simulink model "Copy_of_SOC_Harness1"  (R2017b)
settings: Solver=FixedStepDiscrete  StartTime=0.0  StopTime=2  FixedStep=0.01  RelTol=1e-3  EnableMultiTasking=on
undefined symbols (not defined in the file): sigbuilder_block

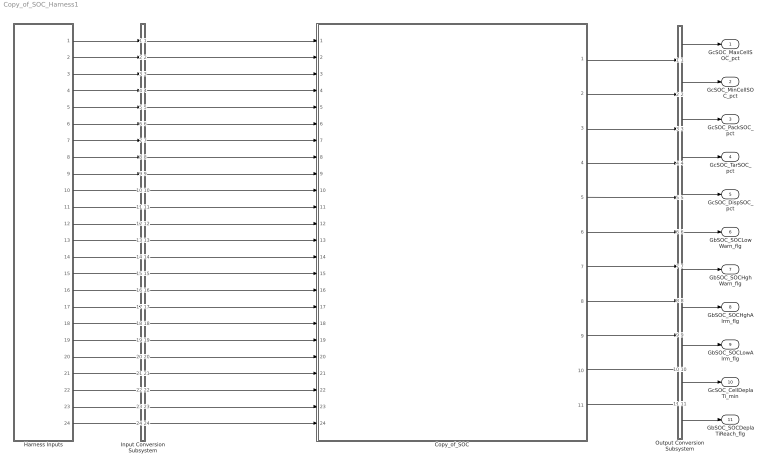
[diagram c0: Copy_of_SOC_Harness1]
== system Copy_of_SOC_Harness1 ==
  Copy_of_SOC : ModelReference  ModelNameDialog=Copy_of_SOC  SimulationMode=Normal  ModelReferenceVersion='M110C113'
  Harness Inputs : Subsystem  Tag=STV Subsys  LoadFcn=sigbuilder_block('load');  StartFcn=sigbuilder_block('start');  StopFcn=sigbuilder_block('stop');  ClipboardFcn=sigbuilder_block('clipboard');  mask(Sigbuilder block){tuvar=[0:10]}
      mask init:
      | if ~strcmp(get_param(bdroot(gcb),'SimulationStatus'),'stopped'),tuvar = sigbuilder_block('maskInit'); end
  Input Conversion Subsystem : Subsystem  Tag=__SLT_ICS__  Description=Signal spec. and routing
  Output Conversion Subsystem : Subsystem  Tag=__SLT_OCS__  Description=Signal spec. and routing
  GcSOC_MaxCellSOC_pct : Outport  OutDataTypeStr=single  PortDimensions=[1]
  GcSOC_MinCellSOC_pct : Outport  Port=2  OutDataTypeStr=single  PortDimensions=[1]
  GcSOC_PackSOC_pct : Outport  Port=3  OutDataTypeStr=single  PortDimensions=[1]
  GcSOC_TarSOC_pct : Outport  Port=4  OutDataTypeStr=single  PortDimensions=[1]
  GcSOC_DispSOC_pct : Outport  Port=5  OutDataTypeStr=single  PortDimensions=[1]
  GbSOC_SOCLowWarn_flg : Outport  Port=6  OutDataTypeStr=boolean  PortDimensions=[1]
  GbSOC_SOCHghWarn_flg : Outport  Port=7  OutDataTypeStr=boolean  PortDimensions=[1]
  GbSOC_SOCHghAlrm_flg : Outport  Port=8  OutDataTypeStr=boolean  PortDimensions=[1]
  GbSOC_SOCLowAlrm_flg : Outport  Port=9  OutDataTypeStr=boolean  PortDimensions=[1]
  GcSOC_CellDeplaTi_min : Outport  Port=10  OutDataTypeStr=uint32  PortDimensions=[1]
  GbSOC_SOCDeplaTiReach_flg : Outport  Port=11  OutDataTypeStr=boolean  PortDimensions=[1]
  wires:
  Harness Inputs/1(GcHDP_PackCrnt_A) -> Input Conversion Subsystem/1(Inport_1)
  Harness Inputs/2(GcHDP_PackVolt_V) -> Input Conversion Subsystem/2(Inport_2)
  Harness Inputs/3(GbACC_ACChrgFinish_flg) -> Input Conversion Subsystem/3(Inport_3)
  Harness Inputs/4(GbDCC_DCChrgFinish_flg) -> Input Conversion Subsystem/4(Inport_4)
  Harness Inputs/5(GcRTC_SleepTime_min) -> Input Conversion Subsystem/5(Inport_5)
  Harness Inputs/6(GcCDP_MaxCellVolt_mV) -> Input Conversion Subsystem/6(Inport_6)
  Harness Inputs/7(GcCDP_MinCellVolt_mV) -> Input Conversion Subsystem/7(Inport_7)
  Harness Inputs/8(GcCDP_MinCellTemp_C) -> Input Conversion Subsystem/8(Inport_8)
  Harness Inputs/9(GbCDP_SumCellVoltVld_flg) -> Input Conversion Subsystem/9(Inport_9)
  Harness Inputs/10(GeMSM_BMUState_enum) -> Input Conversion Subsystem/10(Inport_10)
  Harness Inputs/11(GbNDP_ReadMaxCellSOCVld_flg) -> Input Conversion Subsystem/11(Inport_11)
  Harness Inputs/12(GbNDP_ReadMinCellSOCVld_flg) -> Input Conversion Subsystem/12(Inport_12)
  Harness Inputs/13(GbNDP_ReadMaxCellVoltVld_flg) -> Input Conversion Subsystem/13(Inport_13)
  Harness Inputs/14(GbNDP_ReadMinCellVoltVld_flg) -> Input Conversion Subsystem/14(Inport_14)
  Harness Inputs/15(GcSOH_CurrBatCap_Ah) -> Input Conversion Subsystem/15(Inport_15)
  Harness Inputs/16(GbUDS_MnlSOCCorrd_flg) -> Input Conversion Subsystem/16(Inport_16)
  Harness Inputs/17(GeCTC_CtrCtlConnMode_enum) -> Input Conversion Subsystem/17(Inport_17)
  Harness Inputs/18(GbNDP_ReadDispSOCVld_flg) -> Input Conversion Subsystem/18(Inport_18)
  Harness Inputs/19(GbHDP_PackCrntVld_flg) -> Input Conversion Subsystem/19(Inport_19)
  Harness Inputs/20(GbDCC_ChrgSt2StepChrg_flg) -> Input Conversion Subsystem/20(Inport_20)
  Harness Inputs/21(GbACC_ChrgSt2StepChrg_flg) -> Input Conversion Subsystem/21(Inport_21)
  Harness Inputs/22(GcADP_YearSet_Yr) -> Input Conversion Subsystem/22(Inport_22)
  Harness Inputs/23(GbISP_TF37FTiout_flg) -> Input Conversion Subsystem/23(Inport_23)
  Harness Inputs/24(GeUDS_CapSel_enum) -> Input Conversion Subsystem/24(Inport_24)
  Output Conversion Subsystem/1(Outport_1) -> GcSOC_MaxCellSOC_pct/1
  Output Conversion Subsystem/2(Outport_2) -> GcSOC_MinCellSOC_pct/1
  Output Conversion Subsystem/3(Outport_3) -> GcSOC_PackSOC_pct/1
  Output Conversion Subsystem/4(Outport_4) -> GcSOC_TarSOC_pct/1
  Output Conversion Subsystem/5(Outport_5) -> GcSOC_DispSOC_pct/1
  Output Conversion Subsystem/6(Outport_6) -> GbSOC_SOCLowWarn_flg/1
  Output Conversion Subsystem/7(Outport_7) -> GbSOC_SOCHghWarn_flg/1
  Output Conversion Subsystem/8(Outport_8) -> GbSOC_SOCHghAlrm_flg/1
  Output Conversion Subsystem/9(Outport_9) -> GbSOC_SOCLowAlrm_flg/1
  Output Conversion Subsystem/10(Outport_10) -> GcSOC_CellDeplaTi_min/1
  Output Conversion Subsystem/11(Outport_11) -> GbSOC_SOCDeplaTiReach_flg/1
  Input Conversion Subsystem/1(Outport_1) -> Copy_of_SOC/1
  Input Conversion Subsystem/2(Outport_2) -> Copy_of_SOC/2
  Input Conversion Subsystem/3(Outport_3) -> Copy_of_SOC/3
  Input Conversion Subsystem/4(Outport_4) -> Copy_of_SOC/4
  Input Conversion Subsystem/5(Outport_5) -> Copy_of_SOC/5
  Input Conversion Subsystem/6(Outport_6) -> Copy_of_SOC/6
  Input Conversion Subsystem/7(Outport_7) -> Copy_of_SOC/7
  Input Conversion Subsystem/8(Outport_8) -> Copy_of_SOC/8
  Input Conversion Subsystem/9(Outport_9) -> Copy_of_SOC/9
  Input Conversion Subsystem/10(Outport_10) -> Copy_of_SOC/10
  Input Conversion Subsystem/11(Outport_11) -> Copy_of_SOC/11
  Input Conversion Subsystem/12(Outport_12) -> Copy_of_SOC/12
  Input Conversion Subsystem/13(Outport_13) -> Copy_of_SOC/13
  Input Conversion Subsystem/14(Outport_14) -> Copy_of_SOC/14
  Input Conversion Subsystem/15(Outport_15) -> Copy_of_SOC/15
  Input Conversion Subsystem/16(Outport_16) -> Copy_of_SOC/16
  Input Conversion Subsystem/17(Outport_17) -> Copy_of_SOC/17
  Input Conversion Subsystem/18(Outport_18) -> Copy_of_SOC/18
  Input Conversion Subsystem/19(Outport_19) -> Copy_of_SOC/19
  Input Conversion Subsystem/20(Outport_20) -> Copy_of_SOC/20
  Input Conversion Subsystem/21(Outport_21) -> Copy_of_SOC/21
  Input Conversion Subsystem/22(Outport_22) -> Copy_of_SOC/22
  Input Conversion Subsystem/23(Outport_23) -> Copy_of_SOC/23
  Input Conversion Subsystem/24(Outport_24) -> Copy_of_SOC/24
  Copy_of_SOC/1 -> Output Conversion Subsystem/1(Inport_1)
  Copy_of_SOC/2 -> Output Conversion Subsystem/2(Inport_2)
  Copy_of_SOC/3 -> Output Conversion Subsystem/3(Inport_3)
  Copy_of_SOC/4 -> Output Conversion Subsystem/4(Inport_4)
  Copy_of_SOC/5 -> Output Conversion Subsystem/5(Inport_5)
  Copy_of_SOC/6 -> Output Conversion Subsystem/6(Inport_6)
  Copy_of_SOC/7 -> Output Conversion Subsystem/7(Inport_7)
  Copy_of_SOC/8 -> Output Conversion Subsystem/8(Inport_8)
  Copy_of_SOC/9 -> Output Conversion Subsystem/9(Inport_9)
  Copy_of_SOC/10 -> Output Conversion Subsystem/10(Inport_10)
  Copy_of_SOC/11 -> Output Conversion Subsystem/11(Inport_11)

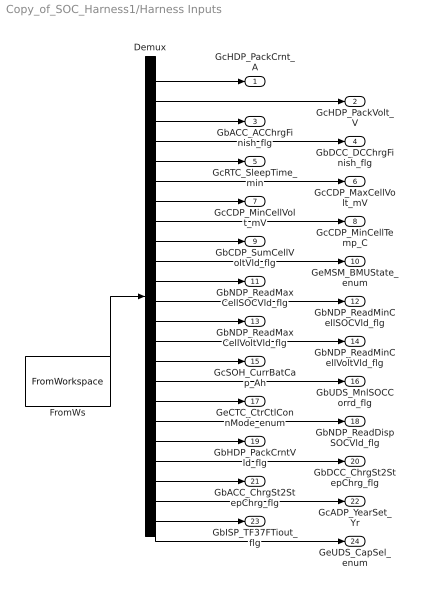
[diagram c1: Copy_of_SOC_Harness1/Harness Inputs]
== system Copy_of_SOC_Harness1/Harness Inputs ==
  Demux : Demux  Tag=STV Demux  Outputs=24
  FromWs : FromWorkspace  Tag=STV FromWs  VariableName=tuvar  SampleTime=0
  GcHDP_PackCrnt_A : Outport  Tag=STV Outport
  GcHDP_PackVolt_V : Outport  Tag=STV Outport  Port=2
  GbACC_ACChrgFinish_flg : Outport  Tag=STV Outport  Port=3
  GbDCC_DCChrgFinish_flg : Outport  Tag=STV Outport  Port=4
  GcRTC_SleepTime_min : Outport  Tag=STV Outport  Port=5
  GcCDP_MaxCellVolt_mV : Outport  Tag=STV Outport  Port=6
  GcCDP_MinCellVolt_mV : Outport  Tag=STV Outport  Port=7
  GcCDP_MinCellTemp_C : Outport  Tag=STV Outport  Port=8
  GbCDP_SumCellVoltVld_flg : Outport  Tag=STV Outport  Port=9
  GeMSM_BMUState_enum : Outport  Tag=STV Outport  Port=10
  GbNDP_ReadMaxCellSOCVld_flg : Outport  Tag=STV Outport  Port=11
  GbNDP_ReadMinCellSOCVld_flg : Outport  Tag=STV Outport  Port=12
  GbNDP_ReadMaxCellVoltVld_flg : Outport  Tag=STV Outport  Port=13
  GbNDP_ReadMinCellVoltVld_flg : Outport  Tag=STV Outport  Port=14
  GcSOH_CurrBatCap_Ah : Outport  Tag=STV Outport  Port=15
  GbUDS_MnlSOCCorrd_flg : Outport  Tag=STV Outport  Port=16
  GeCTC_CtrCtlConnMode_enum : Outport  Tag=STV Outport  Port=17
  GbNDP_ReadDispSOCVld_flg : Outport  Tag=STV Outport  Port=18
  GbHDP_PackCrntVld_flg : Outport  Tag=STV Outport  Port=19
  GbDCC_ChrgSt2StepChrg_flg : Outport  Tag=STV Outport  Port=20
  GbACC_ChrgSt2StepChrg_flg : Outport  Tag=STV Outport  Port=21
  GcADP_YearSet_Yr : Outport  Tag=STV Outport  Port=22
  GbISP_TF37FTiout_flg : Outport  Tag=STV Outport  Port=23
  GeUDS_CapSel_enum : Outport  Tag=STV Outport  Port=24
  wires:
  FromWs/1 -> Demux/1
  Demux/1 -> GcHDP_PackCrnt_A/1
  Demux/2 -> GcHDP_PackVolt_V/1
  Demux/3 -> GbACC_ACChrgFinish_flg/1
  Demux/4 -> GbDCC_DCChrgFinish_flg/1
  Demux/5 -> GcRTC_SleepTime_min/1
  Demux/6 -> GcCDP_MaxCellVolt_mV/1
  Demux/7 -> GcCDP_MinCellVolt_mV/1
  Demux/8 -> GcCDP_MinCellTemp_C/1
  Demux/9 -> GbCDP_SumCellVoltVld_flg/1
  Demux/10 -> GeMSM_BMUState_enum/1
  Demux/11 -> GbNDP_ReadMaxCellSOCVld_flg/1
  Demux/12 -> GbNDP_ReadMinCellSOCVld_flg/1
  Demux/13 -> GbNDP_ReadMaxCellVoltVld_flg/1
  Demux/14 -> GbNDP_ReadMinCellVoltVld_flg/1
  Demux/15 -> GcSOH_CurrBatCap_Ah/1
  Demux/16 -> GbUDS_MnlSOCCorrd_flg/1
  Demux/17 -> GeCTC_CtrCtlConnMode_enum/1
  Demux/18 -> GbNDP_ReadDispSOCVld_flg/1
  Demux/19 -> GbHDP_PackCrntVld_flg/1
  Demux/20 -> GbDCC_ChrgSt2StepChrg_flg/1
  Demux/21 -> GbACC_ChrgSt2StepChrg_flg/1
  Demux/22 -> GcADP_YearSet_Yr/1
  Demux/23 -> GbISP_TF37FTiout_flg/1
  Demux/24 -> GeUDS_CapSel_enum/1

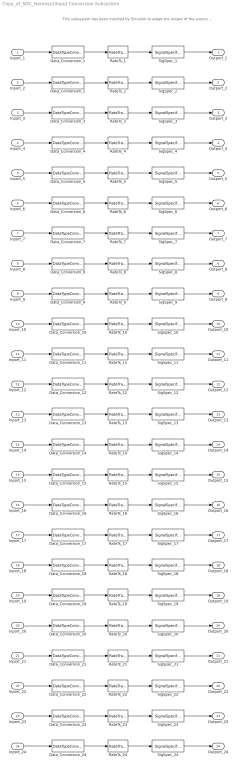
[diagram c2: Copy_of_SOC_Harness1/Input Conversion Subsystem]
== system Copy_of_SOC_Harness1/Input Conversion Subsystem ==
  note: This subsystem has been inserted by Simulink to adapt the output of the source blocks to the interface required by the harnessed component. Modifying the contents of this subsystem may result in compilation and simulation failure.
  Inport_1 : Inport
  Inport_2 : Inport  Port=2
  Inport_3 : Inport  Port=3
  Inport_4 : Inport  Port=4
  Inport_5 : Inport  Port=5
  Inport_6 : Inport  Port=6
  Inport_7 : Inport  Port=7
  Inport_8 : Inport  Port=8
  Inport_9 : Inport  Port=9
  Inport_10 : Inport  Port=10
  Inport_11 : Inport  Port=11
  Inport_12 : Inport  Port=12
  Inport_13 : Inport  Port=13
  Inport_14 : Inport  Port=14
  Inport_15 : Inport  Port=15
  Inport_16 : Inport  Port=16
  Inport_17 : Inport  Port=17
  Inport_18 : Inport  Port=18
  Inport_19 : Inport  Port=19
  Inport_20 : Inport  Port=20
  Inport_21 : Inport  Port=21
  Inport_22 : Inport  Port=22
  Inport_23 : Inport  Port=23
  Inport_24 : Inport  Port=24
  Data_Conversion_{1..2,8,15} (4 alike) : DataTypeConversion  OutDataTypeStr=single
  Data_Conversion_10 : DataTypeConversion  OutDataTypeStr=uint8
  Data_Conversion_{3..4,9,11..14,16,18..21,23} (13 alike) : DataTypeConversion  OutDataTypeStr=boolean
  Data_Conversion_17 : DataTypeConversion  OutDataTypeStr=uint8
  Data_Conversion_22 : DataTypeConversion  OutDataTypeStr=uint16
  Data_Conversion_24 : DataTypeConversion  OutDataTypeStr=uint8
  Data_Conversion_5 : DataTypeConversion  OutDataTypeStr=uint32
  Data_Conversion_6 : DataTypeConversion  OutDataTypeStr=uint16
  Data_Conversion_7 : DataTypeConversion  OutDataTypeStr=uint16
  RateTs_{1..24} (24 alike) : RateTransition  OutPortSampleTime=0.01
  SigSpec_1 : SignalSpecification  OutDataTypeStr=single  Unit=A  Dimensions=[1]  SampleTime=0.01
  SigSpec_10 : SignalSpecification  OutDataTypeStr=uint8  Unit=enum  Dimensions=[1]  SampleTime=0.01
  SigSpec_{3..4,9,11..14,16,18..21,23} (13 alike) : SignalSpecification  OutDataTypeStr=boolean  Unit=flag  Dimensions=[1]  SampleTime=0.01
  SigSpec_15 : SignalSpecification  OutDataTypeStr=single  Unit=Ah  Dimensions=[1]  SampleTime=0.01
  SigSpec_17 : SignalSpecification  OutDataTypeStr=uint8  Unit=enum  Dimensions=[1]  SampleTime=0.01
  SigSpec_2 : SignalSpecification  OutDataTypeStr=single  Unit=V  Dimensions=[1]  SampleTime=0.01
  SigSpec_22 : SignalSpecification  OutDataTypeStr=uint16  Unit=Yr  Dimensions=[1]  SampleTime=0.01
  SigSpec_24 : SignalSpecification  OutDataTypeStr=uint8  Unit=numb  Dimensions=[1]  SampleTime=0.01
  SigSpec_5 : SignalSpecification  OutDataTypeStr=uint32  Unit=min  Dimensions=[1]  SampleTime=0.01
  SigSpec_6 : SignalSpecification  OutDataTypeStr=uint16  Unit=mV  Dimensions=[1]  SampleTime=0.01
  SigSpec_7 : SignalSpecification  OutDataTypeStr=uint16  Unit=mV  Dimensions=[1]  SampleTime=0.01
  SigSpec_8 : SignalSpecification  OutDataTypeStr=single  Unit=C  Dimensions=[1]  SampleTime=0.01
  Outport_1 : Outport
  Outport_2 : Outport  Port=2
  Outport_3 : Outport  Port=3
  Outport_4 : Outport  Port=4
  Outport_5 : Outport  Port=5
  Outport_6 : Outport  Port=6
  Outport_7 : Outport  Port=7
  Outport_8 : Outport  Port=8
  Outport_9 : Outport  Port=9
  Outport_10 : Outport  Port=10
  Outport_11 : Outport  Port=11
  Outport_12 : Outport  Port=12
  Outport_13 : Outport  Port=13
  Outport_14 : Outport  Port=14
  Outport_15 : Outport  Port=15
  Outport_16 : Outport  Port=16
  Outport_17 : Outport  Port=17
  Outport_18 : Outport  Port=18
  Outport_19 : Outport  Port=19
  Outport_20 : Outport  Port=20
  Outport_21 : Outport  Port=21
  Outport_22 : Outport  Port=22
  Outport_23 : Outport  Port=23
  Outport_24 : Outport  Port=24
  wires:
  SigSpec_1/1 -> Outport_1/1
  RateTs_1/1 -> SigSpec_1/1
  Data_Conversion_1/1 -> RateTs_1/1
  Inport_1/1 -> Data_Conversion_1/1
  SigSpec_2/1 -> Outport_2/1
  RateTs_2/1 -> SigSpec_2/1
  Data_Conversion_2/1 -> RateTs_2/1
  Inport_2/1 -> Data_Conversion_2/1
  SigSpec_3/1 -> Outport_3/1
  RateTs_3/1 -> SigSpec_3/1
  Data_Conversion_3/1 -> RateTs_3/1
  Inport_3/1 -> Data_Conversion_3/1
  SigSpec_4/1 -> Outport_4/1
  RateTs_4/1 -> SigSpec_4/1
  Data_Conversion_4/1 -> RateTs_4/1
  Inport_4/1 -> Data_Conversion_4/1
  SigSpec_5/1 -> Outport_5/1
  RateTs_5/1 -> SigSpec_5/1
  Data_Conversion_5/1 -> RateTs_5/1
  Inport_5/1 -> Data_Conversion_5/1
  SigSpec_6/1 -> Outport_6/1
  RateTs_6/1 -> SigSpec_6/1
  Data_Conversion_6/1 -> RateTs_6/1
  Inport_6/1 -> Data_Conversion_6/1
  SigSpec_7/1 -> Outport_7/1
  RateTs_7/1 -> SigSpec_7/1
  Data_Conversion_7/1 -> RateTs_7/1
  Inport_7/1 -> Data_Conversion_7/1
  SigSpec_8/1 -> Outport_8/1
  RateTs_8/1 -> SigSpec_8/1
  Data_Conversion_8/1 -> RateTs_8/1
  Inport_8/1 -> Data_Conversion_8/1
  SigSpec_9/1 -> Outport_9/1
  RateTs_9/1 -> SigSpec_9/1
  Data_Conversion_9/1 -> RateTs_9/1
  Inport_9/1 -> Data_Conversion_9/1
  SigSpec_10/1 -> Outport_10/1
  RateTs_10/1 -> SigSpec_10/1
  Data_Conversion_10/1 -> RateTs_10/1
  Inport_10/1 -> Data_Conversion_10/1
  SigSpec_11/1 -> Outport_11/1
  RateTs_11/1 -> SigSpec_11/1
  Data_Conversion_11/1 -> RateTs_11/1
  Inport_11/1 -> Data_Conversion_11/1
  SigSpec_12/1 -> Outport_12/1
  RateTs_12/1 -> SigSpec_12/1
  Data_Conversion_12/1 -> RateTs_12/1
  Inport_12/1 -> Data_Conversion_12/1
  SigSpec_13/1 -> Outport_13/1
  RateTs_13/1 -> SigSpec_13/1
  Data_Conversion_13/1 -> RateTs_13/1
  Inport_13/1 -> Data_Conversion_13/1
  SigSpec_14/1 -> Outport_14/1
  RateTs_14/1 -> SigSpec_14/1
  Data_Conversion_14/1 -> RateTs_14/1
  Inport_14/1 -> Data_Conversion_14/1
  SigSpec_15/1 -> Outport_15/1
  RateTs_15/1 -> SigSpec_15/1
  Data_Conversion_15/1 -> RateTs_15/1
  Inport_15/1 -> Data_Conversion_15/1
  SigSpec_16/1 -> Outport_16/1
  RateTs_16/1 -> SigSpec_16/1
  Data_Conversion_16/1 -> RateTs_16/1
  Inport_16/1 -> Data_Conversion_16/1
  SigSpec_17/1 -> Outport_17/1
  RateTs_17/1 -> SigSpec_17/1
  Data_Conversion_17/1 -> RateTs_17/1
  Inport_17/1 -> Data_Conversion_17/1
  SigSpec_18/1 -> Outport_18/1
  RateTs_18/1 -> SigSpec_18/1
  Data_Conversion_18/1 -> RateTs_18/1
  Inport_18/1 -> Data_Conversion_18/1
  SigSpec_19/1 -> Outport_19/1
  RateTs_19/1 -> SigSpec_19/1
  Data_Conversion_19/1 -> RateTs_19/1
  Inport_19/1 -> Data_Conversion_19/1
  SigSpec_20/1 -> Outport_20/1
  RateTs_20/1 -> SigSpec_20/1
  Data_Conversion_20/1 -> RateTs_20/1
  Inport_20/1 -> Data_Conversion_20/1
  SigSpec_21/1 -> Outport_21/1
  RateTs_21/1 -> SigSpec_21/1
  Data_Conversion_21/1 -> RateTs_21/1
  Inport_21/1 -> Data_Conversion_21/1
  SigSpec_22/1 -> Outport_22/1
  RateTs_22/1 -> SigSpec_22/1
  Data_Conversion_22/1 -> RateTs_22/1
  Inport_22/1 -> Data_Conversion_22/1
  SigSpec_23/1 -> Outport_23/1
  RateTs_23/1 -> SigSpec_23/1
  Data_Conversion_23/1 -> RateTs_23/1
  Inport_23/1 -> Data_Conversion_23/1
  SigSpec_24/1 -> Outport_24/1
  RateTs_24/1 -> SigSpec_24/1
  Data_Conversion_24/1 -> RateTs_24/1
  Inport_24/1 -> Data_Conversion_24/1

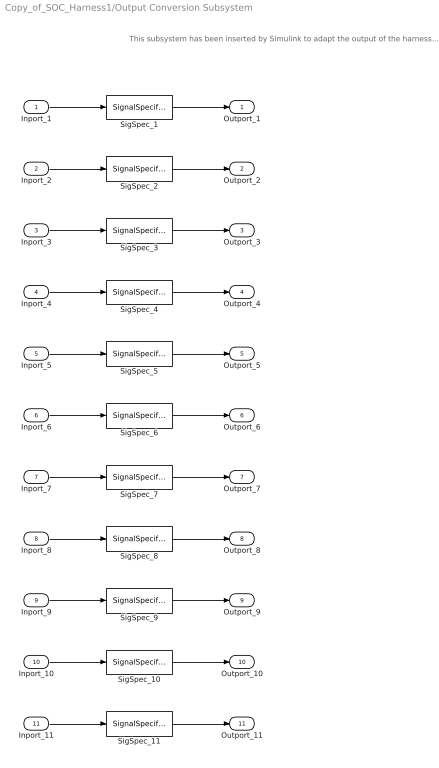
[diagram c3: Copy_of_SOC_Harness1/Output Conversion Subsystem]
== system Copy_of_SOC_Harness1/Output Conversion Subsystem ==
  note: This subsystem has been inserted by Simulink to adapt the output of the harnessed component to the interface required by the sink blocks. Modifying the contents of this subsystem may result in compilation and simulation failure.
  Inport_1 : Inport
  Inport_2 : Inport  Port=2
  Inport_3 : Inport  Port=3
  Inport_4 : Inport  Port=4
  Inport_5 : Inport  Port=5
  Inport_6 : Inport  Port=6
  Inport_7 : Inport  Port=7
  Inport_8 : Inport  Port=8
  Inport_9 : Inport  Port=9
  Inport_10 : Inport  Port=10
  Inport_11 : Inport  Port=11
  SigSpec_{1..5} (5 alike) : SignalSpecification  OutDataTypeStr=single  Unit=pct  Dimensions=[1]  SampleTime=0.01
  SigSpec_10 : SignalSpecification  OutDataTypeStr=uint32  Unit=min  Dimensions=[1]  SampleTime=0.01
  SigSpec_11 : SignalSpecification  OutDataTypeStr=boolean  Unit=flg  Dimensions=[1]  SampleTime=0.01
  SigSpec_{6..9} (4 alike) : SignalSpecification  OutDataTypeStr=boolean  Unit=flag  Dimensions=[1]  SampleTime=0.01
  Outport_1 : Outport
  Outport_2 : Outport  Port=2
  Outport_3 : Outport  Port=3
  Outport_4 : Outport  Port=4
  Outport_5 : Outport  Port=5
  Outport_6 : Outport  Port=6
  Outport_7 : Outport  Port=7
  Outport_8 : Outport  Port=8
  Outport_9 : Outport  Port=9
  Outport_10 : Outport  Port=10
  Outport_11 : Outport  Port=11
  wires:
  Inport_1/1 -> SigSpec_1/1
  SigSpec_1/1 -> Outport_1/1
  Inport_2/1 -> SigSpec_2/1
  SigSpec_2/1 -> Outport_2/1
  Inport_3/1 -> SigSpec_3/1
  SigSpec_3/1 -> Outport_3/1
  Inport_4/1 -> SigSpec_4/1
  SigSpec_4/1 -> Outport_4/1
  Inport_5/1 -> SigSpec_5/1
  SigSpec_5/1 -> Outport_5/1
  Inport_6/1 -> SigSpec_6/1
  SigSpec_6/1 -> Outport_6/1
  Inport_7/1 -> SigSpec_7/1
  SigSpec_7/1 -> Outport_7/1
  Inport_8/1 -> SigSpec_8/1
  SigSpec_8/1 -> Outport_8/1
  Inport_9/1 -> SigSpec_9/1
  SigSpec_9/1 -> Outport_9/1
  Inport_10/1 -> SigSpec_10/1
  SigSpec_10/1 -> Outport_10/1
  Inport_11/1 -> SigSpec_11/1
  SigSpec_11/1 -> Outport_11/1
